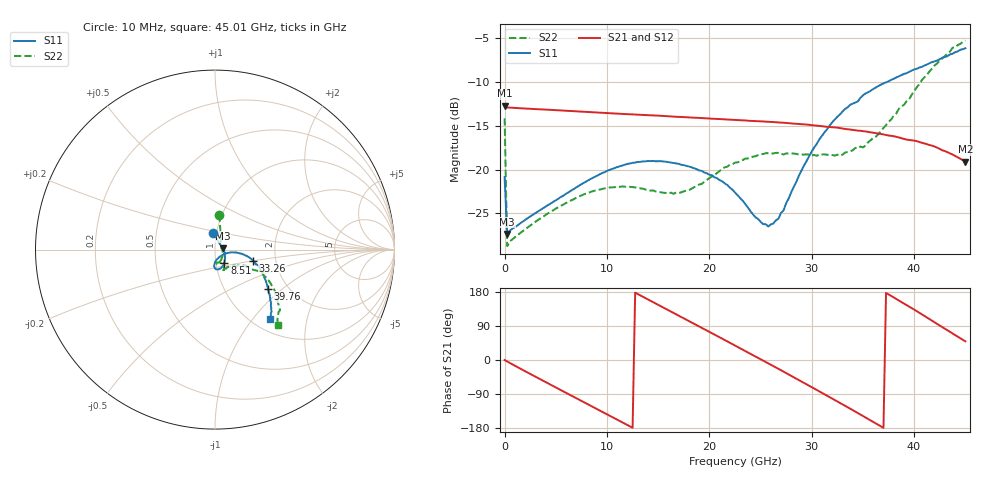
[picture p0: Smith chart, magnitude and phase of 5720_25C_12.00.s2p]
! Device:  ADRF5720
! Description: 0.5dB LSB GaAs MMIC 6-bit Digital Attenuator
! Frequency:  0.000009 -  40 GHz
! Ports:
!	RF1	= Port 1
!	RF2	= Port 2
! Vdd:  3.3 Volt
! Vss:  -3.3 Volt
! Control:  0/3.3 Volt
! State:  12.00 dB attenuation
! Data:  The device was measured using G-S-G Probes on a matrix board.
!  Data was collected using an calibrated 4 port network analyzer.
!  The reference plane for this measurement is at the launchers.
! Note:  Analog Devices supplies this data as a sample of measured data
!  for this product.  Your particular data for this product may vary.
!  Data was taken at 25 degrees C.
!  Analog Devices reserves the right to change this data at anytime.
# GHZ S DB R 45.0
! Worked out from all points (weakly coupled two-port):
!   181 points, 10 MHz to 45.01 GHz, reference 45 ohm
!   highest |S21| = -12.73 dB at 10 MHz (marker M1); lowest = -19.1 dB at 45.01 GHz (marker M2)
!   lowest |S11| = -27.4 dB at 260 MHz (marker M3), VSWR 1.09, Z = 48.9 + j0.782 ohm
!   |S11| at or under -10 dB: start of sweep to 37.37 GHz
!   |S22| runs from -28.8 to -5.3 dB; largest |S21 - S12| = 0.0003
!   S11 on the Smith chart (normalised r, x): 10 MHz: 0.97, +0.18; 8.51 GHz: 1.10, -0.16; 33.26 GHz: 1.53, -0.20; 39.76 GHz: 1.59, -0.80; 45.01 GHz: 1.20, -1.22
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0.01  -20.85 96.1  -12.73 -0.2  -12.73 -0.2  -14.15 82.8
0.26  -27.37 10.7  -12.92 -4.0  -12.92 -4.0  -28.75 11.2
2.26  -25.55 -12.1  -13.05 -33.1  -13.06 -33.1  -26.61 -21.6
4.26  -24.06 -28.6  -13.18 -61.7  -13.18 -61.7  -25.00 -43.3
7.76  -21.51 -50.1  -13.41 -111.5  -13.41 -111.5  -22.83 -67.3
8.51  -21.02 -54.2  -13.46 -122.1  -13.46 -122.1  -22.52 -71.2
12.01  -19.36 -71.4  -13.68 -171.7  -13.68 -171.7  -21.99 -83.1
15.26  -19.05 -83.5  -13.87 142.0  -13.87 142.1  -22.60 -82.7
17.01  -19.35 -88.4  -13.99 117.1  -14.00 117.2  -22.67 -75.7
19.01  -20.11 -91.6  -14.11 88.5  -14.12 88.6  -21.71 -66.4
21.26  -21.34 -92.6  -14.26 56.3  -14.26 56.3  -19.93 -62.9
22.76  -22.94 -90.4  -14.36 34.7  -14.36 34.7  -19.18 -63.1
25.26  -26.23 -63.9  -14.52 -1.5  -14.52 -1.5  -18.24 -66.4
26.26  -26.16 -42.2  -14.58 -16.1  -14.59 -16.1  -18.16 -66.0
27.26  -24.65 -23.1  -14.66 -30.9  -14.67 -30.8  -18.28 -66.9
30.26  -17.46 -8.1  -14.96 -75.5  -14.96 -75.4  -18.34 -63.5
33.26  -13.09 -16.2  -15.37 -120.9  -15.37 -120.8  -18.06 -50.8
35.01  -11.53 -21.5  -15.62 -147.6  -15.62 -147.5  -17.48 -42.3
37.76  -9.76 -30.7  -16.16 169.2  -16.16 169.3  -14.30 -27.9
39.76  -8.71 -36.5  -16.66 137.2  -16.66 137.3  -11.48 -26.4
42.51  -7.41 -43.1  -17.65 90.6  -17.65 90.7  -7.56 -36.1
45.01  -6.16 -51.6  -19.09 49.2  -19.09 49.3  -5.27 -50.3
